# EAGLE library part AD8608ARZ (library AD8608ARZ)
Precision, Low Noise, CMOS, Rail-to-Rail, Input/Output Operational Amplifiers Check availability
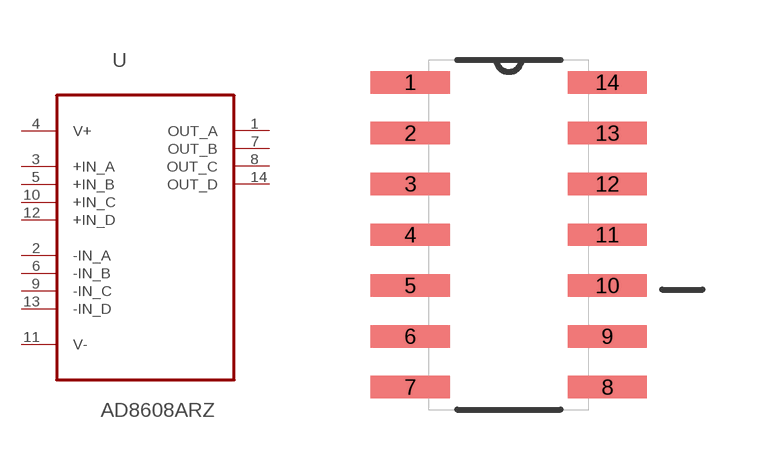
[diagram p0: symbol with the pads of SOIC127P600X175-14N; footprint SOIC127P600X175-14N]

Designator prefix U

## AD8608ARZ (Availability: In Stock; Description: CMOS Amplifier 4 Circuit Rail-to-Rail 14-SOIC; MF: Analog Devices; MP: AD8608ARZ-REEL7; Package: SOIC-14 Analog Devices; Price: None; Purchase-URL: https://pricing.snapeda.com/search/part/AD8608ARZ-REEL7/?ref=eda)  [SOIC127P600X175-14N]
1  OUT_A  out
2  -IN_A  in
3  +IN_A  in
4  V+  pwr
5  +IN_B  in
6  -IN_B  in
7  OUT_B  out
8  OUT_C  out
9  -IN_C  in
10  +IN_C  in
11  V-  pwr
12  +IN_D  in
13  -IN_D  in
14  OUT_D  out

## Footprint SOIC127P600X175-14N (pad centres in mm)
smd 1.981 x 0.559: 1 -2.464,3.81; 2 -2.464,2.54; 3 -2.464,1.27; 4 -2.464,0; 5 -2.464,-1.27; 6 -2.464,-2.54; 7 -2.464,-3.81; 8 2.464,-3.81; 9 2.464,-2.54; 10 2.464,-1.27; 11 2.464,0; 12 2.464,1.27; 13 2.464,2.54; 14 2.464,3.81

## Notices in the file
This work is licensed under a Creative Commons Attribution-ShareAlike 4.0 International License (CC BY-SA) with Design Exception 1.0
